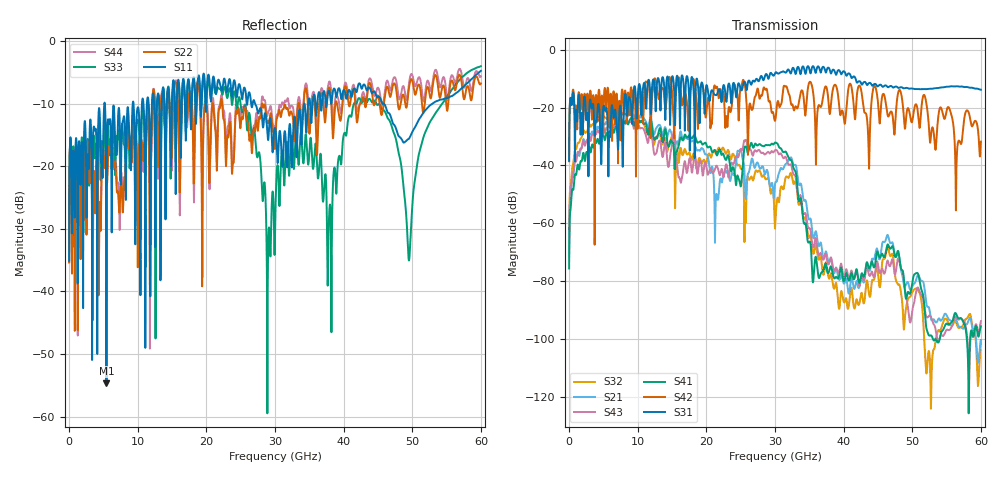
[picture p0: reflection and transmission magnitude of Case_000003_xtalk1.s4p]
! Info: Touchstone file created by circ.  Input file=CasetestDOE_NRZ_template_000003.circ
# Hz S RI R 50
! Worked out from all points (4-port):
!   6000 points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, 10 MHz to 60 GHz, reference 50 ohm
!   strongest paths, dB at 10 MHz, 15.01 GHz, 30.01 GHz, 45.01 GHz, 60 GHz:
!     S31: -38.4, -9.4, -8.2, -12.6, -13.8
!     S42: -38.6, -14.8, -24.6, -18.3, -31.8
!     S41: -75.6, -32.0, -32.1, -70.2, -95.6
!     S43: -71.7, -32.3, -34.7, -74.2, -93.9
!     S21: -71.4, -29.9, -46.5, -70.4, -100.5
!     S32: -68.2, -29.6, -61.7, -77.1, -100.4
!   lowest |S11| = -54.7 dB at 5.45 GHz (marker M1), VSWR 1.00, Z = 49.8 - j0.0605 ohm
!   |S11| at or under -10 dB: start of sweep to 5.141 GHz; 27.09 GHz to 34.25 GHz (7.164 GHz wide, 23.4 % of centre); 45.62 GHz to 52.95 GHz (7.324 GHz wide, 14.9 % of centre)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
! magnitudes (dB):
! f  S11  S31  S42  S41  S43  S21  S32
! 10 MHz  -35.1  -38.4  -38.6  -75.6  -71.7  -71.4  -68.2
! 1.08 GHz  -16.1  -21.6  -20.7  -42.7  -38.1  -37.1  -34.1
! 5.45 GHz  -54.7  -20.2  -20.5  -28.9  -27.0  -25.0  -23.7
! 30.19 GHz  -15.4  -7.8  -21.4  -32.2  -34.7  -45.7  -54.5
! 35.59 GHz  -8.9  -5.8  -15.4  -79.7  -68.4  -65.1  -70.6
! 49.53 GHz  -15.6  -13.5  -20.9  -84.3  -92.3  -81.8  -85.7
! 60 GHz  -4.8  -13.8  -31.8  -95.6  -93.9  -100.5  -100.4
